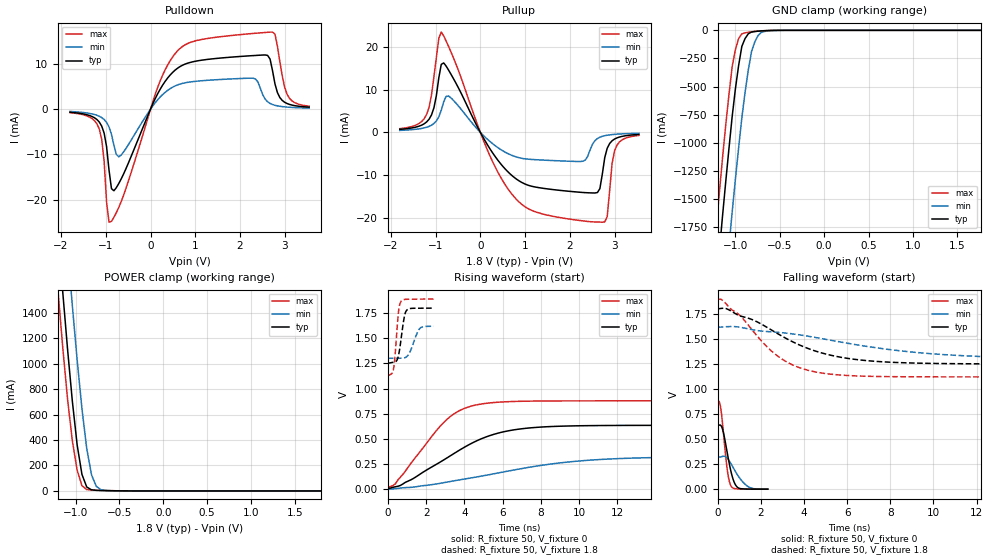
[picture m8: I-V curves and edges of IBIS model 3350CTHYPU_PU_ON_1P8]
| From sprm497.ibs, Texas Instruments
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|   Model Cell 3350CTHYPU_PU_ON_1P8
|BC3350CTHYPU_PU_ON_1P8
[Model]   3350CTHYPU_PU_ON_1P8
Model_type   I/O
Polarity   Non-Inverting
Enable   Active-Low
Vinl =  0.63
Vinh =  1.17
Cref =  15.0000pF
Rref =  100.0000M
Vref =  0V
Vmeas =  0.9
C_comp   1.505312p   1.488461p   1.520888p
[Model Spec]
Vinl   0.63   0.567   0.6615
Vinh   1.17   1.053   1.2285
[Temperature Range]   25   125   -40
[Voltage Range]   1.8   1.62   1.89
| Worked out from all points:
|   slope of the pulldown table from 0 to 0.27 V, typ, clamps not added: 51 ohm
|   slope of the pullup table from 0 to 0.27 V, typ, clamps not added: 57.1 ohm
|   GND clamp passes 1 mA (typ) near -0.58 V on its own axis
|   POWER clamp passes 1 mA (typ) near -0.52 V on its own axis
|   rising waveform, R_fixture 50, V_fixture 0: 20-80 % time 3.46ns typ, 5.9ns min, 2.22ns max; typ from 0.004 V to 0.634 V
|   rising waveform, R_fixture 50, V_fixture 1.8: 20-80 % time 248ps typ, 386ps min, 190ps max; typ from 1.25 V to 1.8 V
|   falling waveform, R_fixture 50, V_fixture 0: 20-80 % time 353ps typ, 589ps min, 255ps max; typ from 0.635 V to 0.002 V
|   falling waveform, R_fixture 50, V_fixture 1.8: 20-80 % time 3.19ns typ, 5.95ns min, 2.16ns max; typ from 1.8 V to 1.25 V
[POWER_clamp]
|   voltage   I(typ)   I(min)   I(max)
-1.8V     7.656A     8.472A     7.195A
-1.2V     2.026A     2.853A     1.569A
-1.145V   1.557A     2.372A     1.122A
-1.055V   838.8mA    1.603A     501mA
-1.036V   702.9mA    1.453A     391.9mA
-981.8mV  361.4mA    1.029A     163mA
-927.3mV  130.1mA    646.4mA    41.15mA
-872.7mV  30.99mA    333.2mA    10.88mA
-818.2mV  8.555mA    127mA      6.719mA
-763.6mV  4.582mA    35.75mA    5.241mA
-709.1mV  3.338mA    9.346mA    4.067mA
1.8V      62.93pA    6.445nA    992.5fA
[Pulldown]
|   voltage   I(typ)   I(min)   I(max)
-1.8V     -681.9uA   -516.6uA   -765.4uA
-1.145V   -2.846mA   -1.565mA   -4.381mA
-1.036V   -5.312mA   -2.288mA   -11.57mA
-927.3mV  -13.49mA   -3.93mA    -25mA
-872.7mV  -17.58mA   -5.576mA   -24.82mA
-709.1mV  -16.44mA   -10.53mA   -21.73mA
218.2mV   4.45mA     2.706mA    6.292mA
763.6mV   9.932mA    5.814mA    14.18mA
2.291V    11.85mA    6.843mA    16.75mA
2.727V    8.542mA    1.025mA    17.05mA
3.055V    1.241mA    457.6uA    3.265mA
3.545V    447.3uA    243.5uA    654.8uA
[Pullup]
|   voltage   I(typ)   I(min)   I(max)
-1.8V     683.6uA    441.3uA    848.3uA
-1.2V     2.424mA    1.182mA    4.185mA
-1.036V   5.748mA    2.058mA    13.02mA
-872.7mV  15.88mA    5.165mA    23.42mA
-709.1mV  14.53mA    8.476mA    20.05mA
327.3mV   -5.597mA   -3.09mA    -7.989mA
1.091V    -12.45mA   -6.301mA   -17.97mA
2.291V    -14.07mA   -6.77mA    -20.7mA
2.618V    -14.08mA   -1.459mA   -20.97mA
2.782V    -5.909mA   -790.9uA   -20.94mA
3V        -1.582mA   -477.1uA   -4.383mA
3.545V    -498.1uA   -234.4uA   -720.4uA
[GND_clamp]
|   voltage   I(typ)   I(min)   I(max)
-1.8V     -7.797A    -8.671A    -7.298A
-1.218V   -2.297A    -3.197A    -1.772A
-1.182V   -1.974A    -2.871A    -1.452A
-1.145V   -1.654A    -2.548A    -1.137A
-1.073V   -1.052A    -1.92A     -571.9mA
-1.036V   -766.4mA   -1.614A    -322.9mA
-963.6mV  -312.3mA   -1.045A    -73.41mA
-927.3mV  -142mA     -777.3mA   -31.06mA
-854.5mV  -30.48mA   -352.7mA   -17.04mA
-818.2mV  -14.94mA   -188mA     -13.06mA
-709.1mV  -5.17mA    -18.24mA   -4.567mA
1.764V    -1.569uA   4.55uA     -7.468uA
[Ramp]
| variable   typ   min   max
dV/dt_f  0.3340597/3.230891n   0.195273/6.135673n   0.4665823/2.166956n
dV/dt_r  0.3804633/3.469875n   0.1935839/5.951636n   0.5262786/2.240441n
R_load = 50
[Rising Waveform]
R_fixture = 50
V_fixture = 0
V_fixture_min = 0
V_fixture_max = 0
|   time   V(typ)   V(min)   V(max)
0s        3.582mV    35.55uV    14.37mV
393ps     24.03mV    4.892mV    52.9mV
1.305ns   103.1mV    19.92mV    281.4mV
3.003ns   300.1mV    67.33mV    678.1mV
3.681ns   380.3mV    90.06mV    773.7mV
4.503ns   467.4mV    116.8mV    831.8mV
6.123ns   572.9mV    173.8mV    867.9mV
8.055ns   617.6mV    237.4mV    875.9mV
12.47ns   633.4mV    306.6mV    877.4mV
19.74ns   634.2mV    321mV      877.4mV
[Rising Waveform]
R_fixture = 50
V_fixture = 1.8
V_fixture_min = 1.62
V_fixture_max = 1.89
|   time   V(typ)   V(min)   V(max)
0s        1.252V     1.3V       1.126V
225ps     1.259V     1.3V       1.152V
294ps     1.261V     1.3V       1.192V
360ps     1.263V     1.301V     1.29V
555ps     1.327V     1.301V     1.758V
675ps     1.468V     1.301V     1.86V
873ps     1.723V     1.305V     1.885V
1.014ns   1.783V     1.321V     1.887V
1.683ns   1.798V     1.599V     1.888V
2.397ns   1.798V     1.618V     1.889V
[Falling Waveform]
R_fixture = 50
V_fixture = 0
V_fixture_min = 0
V_fixture_max = 0
|   time   V(typ)   V(min)   V(max)
0s        634.5mV    322.8mV    882.4mV
114ps     642.1mV    323.1mV    845.3mV
228ps     599.8mV    329mV      652.9mV
456ps     351.9mV    308.6mV    180.3mV
534ps     262.7mV    285.6mV    86.41mV
621ps     175mV      254.6mV    32.58mV
780ps     64.45mV    194.1mV    7.956mV
963ps     13.82mV    130.3mV    3.885mV
1.524ns   2.361mV    15.28mV    2.276mV
2.325ns   1.795mV    2.039mV    1.601mV
[Falling Waveform]
R_fixture = 50
V_fixture = 1.8
V_fixture_min = 1.62
V_fixture_max = 1.89
|   time   V(typ)   V(min)   V(max)
0s        1.801V     1.619V     1.897V
393ps     1.805V     1.624V     1.853V
1.053ns   1.731V     1.618V     1.731V
2.103ns   1.641V     1.579V     1.464V
2.892ns   1.541V     1.566V     1.314V
3.735ns   1.447V     1.544V     1.219V
4.812ns   1.363V     1.506V     1.162V
7.053ns   1.283V     1.423V     1.128V
10.99ns   1.255V     1.339V     1.123V
22.88ns   1.252V     1.302V     1.123V
